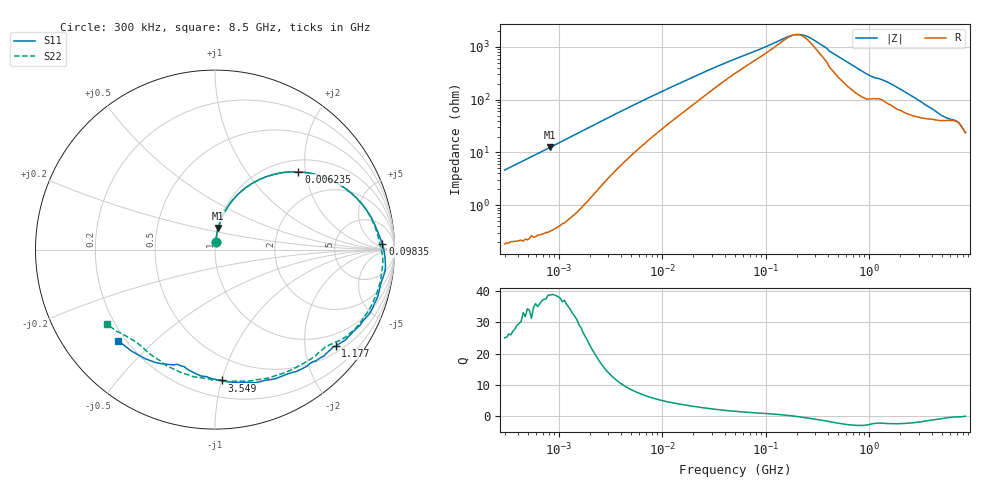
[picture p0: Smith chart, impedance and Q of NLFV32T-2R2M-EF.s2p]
! S-parameter Generated by TDK Corporation
! Copyright(C) 2015 TDK Corporation.
! All Rights Reserved.
! TDK P/N: NLFV32T-2R2M-EF (Inductors)
! Property: L=2.2uH at 7.96MHz
! Size(LxWxT): 3.2x2.5x2.2mm, 0.126x0.098x0.087inches
! Model Type: s2p (Touchstone File Format Version 1.0)
! Frequency: DC=Yes Start=0.3MHz Stop=8500MHz 225points Log-sweep
! Note:
! Model Generated on Jun. 23, 2015
! Hash(MD5):
! Port Assignments:
!  1 ---@@@--- 2
! Applicable Conditions:
!  Temperature = 25 degC
!  DC Bias Current = 0 A
!  Small Signal Operation
! Terms and conditions regarding TDK Simulation Models
! (1)This simulation model is being provided solely for informational purposes. Please refer to the specifications of the products in terms of detailed characteristics of such products.
! (2)In no event shall TDK Corporation of any of its subsidiaries be liable for any loss or damage arising, directly or indirectly,
!  From any information contained in this simulation model, including, but not limited to loss or damages arising from any inaccuracies, omissions or errors in connection with such information.
! (3)Any and all copyrights on this simulation model are owned by TDK Corporation.
!  Duplication or redistribution of this simulation model without prior written permission from TDK Corporation is prohibited.
! (4)This simulation model is subject to any modification or change without any prior notice.
! (5)Neither TDK Corporation nor any of its subsidiaries shall make any warranty, express or implied,
!  Including but not limited to the correctness, implied warranties of merchantability and fitness for a particular purpose with respect to this simulation models.
! (6)The use of this simulation model shall be deemed to have consented to the terms and conditions hereof.
# MHz S MA R 50
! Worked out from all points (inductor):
!   224 points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, 300 kHz to 8.5 GHz, reference 50 ohm
!   read as one part in series: L = 2.45 uH near 314.1 kHz
!   highest Q = 38.7 at 824.8 kHz (marker M1), where L = 2.41 uH
!   self-resonance near 192.9 MHz
!   S11 on the Smith chart (normalised r, x): 300 kHz: 1.00, +0.09; 6.235 MHz: 1.26, +1.83; 98.35 MHz: 24, +11; 1.177 GHz: 0.65, -2.71; 3.549 GHz: 0.32, -1.00; 8.5 GHz: 0.17, -0.39
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0.3  0.04404 85.5  0.9953 -2.6  0.9986 -3.0  0.04396 85.6
0.8248242  0.1215 81.5  0.9888 -7.0  0.9906 -7.4  0.1215 81.5
1.72111  0.2482 73.5  0.9593 -14.4  0.9609 -14.7  0.2484 73.4
3.12867  0.415 61.3  0.8801 -24.4  0.8813 -24.8  0.4153 61.2
6.235074  0.6356 43.0  0.6897 -39.1  0.6905 -39.5  0.6359 42.8
9.430415  0.7418 32.3  0.5466 -46.9  0.5471 -47.3  0.742 32.1
20.60362  0.8597 16.9  0.3124 -55.3  0.3126 -55.7  0.8594 16.7
51.67171  0.9117 6.4  0.1524 -50.9  0.1526 -51.3  0.907 6.1
98.34885  0.9335 1.8  0.09403 -40.2  0.09411 -40.6  0.9222 1.3
195.9978  0.9504 -3.7  0.05553 -2.3  0.05556 -2.7  0.9378 -4.5
235.5662  0.9541 -5.5  0.05725 16.0  0.05729 15.5  0.9378 -6.4
283.1228  0.9539 -7.6  0.06753 30.7  0.0676 30.4  0.9376 -8.6
564.2308  0.9369 -19.4  0.159 48.2  0.159 47.8  0.9226 -21.1
893.5346  0.8953 -30.8  0.2524 39.7  0.2532 38.9  0.8764 -33.6
1177.346  0.8611 -38.7  0.296 27.9  0.2956 27.5  0.8228 -41.2
1551.304  0.8364 -47.8  0.3302 20.8  0.3306 19.9  0.8072 -50.1
2240.89  0.7949 -64.6  0.398 5.3  0.3981 5.1  0.7743 -67.6
3548.748  0.73 -87.1  0.4454 -19.3  0.4466 -20.0  0.7282 -90.6
5126.239  0.6741 -104.7  0.4438 -42.9  0.443 -43.3  0.7035 -109.9
7072.242  0.6997 -114.4  0.3821 -64.3  0.3838 -65.2  0.6851 -133.8
7753.325  0.7219 -122.6  0.3701 -68.0  0.3709 -70.6  0.7136 -140.6
8500  0.7405 -136.7  0.361 -76.2  0.3601 -75.4  0.7313 -145.3
